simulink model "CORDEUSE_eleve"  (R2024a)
settings: Solver=VariableStepAuto  StartTime=0.0  StopTime=10.0  RelTol=1e-3
libraries: fl_lib x15, nesl_utility x4, slpidlib x1

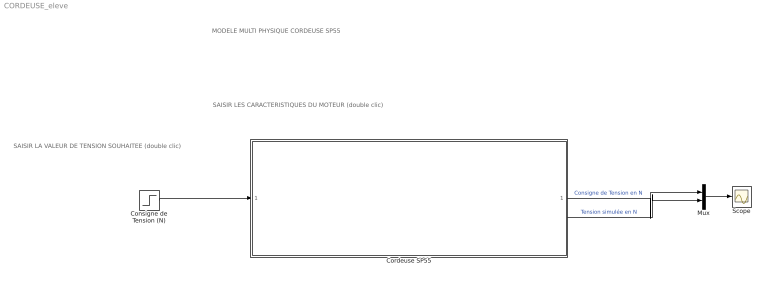
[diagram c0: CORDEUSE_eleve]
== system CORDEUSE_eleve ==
  note: MODELE MULTI PHYSIQUE CORDEUSE SP55
  note: SAISIR LES CARACTERISTIQUES DU MOTEUR (double clic)
  note: SAISIR LA VALEUR DE TENSION SOUHAITEE (double clic)
  Consigne de Tension (N) : Step  After=T  SampleTime=0.001  mask{T=4}
      mask prompts: T "Tension de consigne (en N)"
  Cordeuse SP55 : Subsystem  mask{Kc=0.0001, R=0.0001, L=0.0001}
      mask prompts: Kc "Constante de couple en N.m/A"; R "Résistance induit en ohms."; L "Inductance en mH"
  Mux : Mux  Inputs=2
  Scope : Scope
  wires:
  Mux/1 -> Scope/1
  Consigne de Tension (N)/1 -> Cordeuse SP55/1(In1)
  Cordeuse SP55/1(Consigne) -> Mux/1  "Consigne de Tension en N"
  Cordeuse SP55/2(Tension simulée) -> Mux/2  "Tension simulée en N"

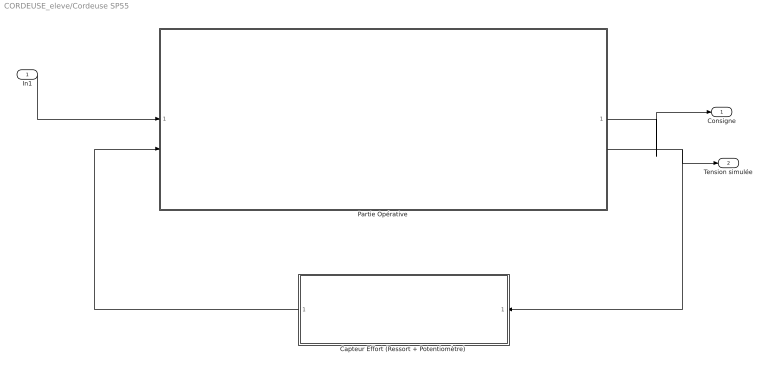
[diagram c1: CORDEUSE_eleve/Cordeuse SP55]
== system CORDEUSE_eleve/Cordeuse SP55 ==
  In1 : Inport
  Capteur Effort (Ressort + Potentiomètre) : Subsystem
  Partie Opérative : Subsystem
  Consigne : Outport
  Tension simulée : Outport  Port=2
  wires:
  Partie Opérative/2(Out2) -> Tension simulée/1, Capteur Effort (Ressort + Potentiomètre)/1(Tension simulée)
  Capteur Effort (Ressort + Potentiomètre)/1(Sortie conditionneur) -> Partie Opérative/2(In1)
  Partie Opérative/1(Out1) -> Consigne/1
  In1/1 -> Partie Opérative/1(In2)

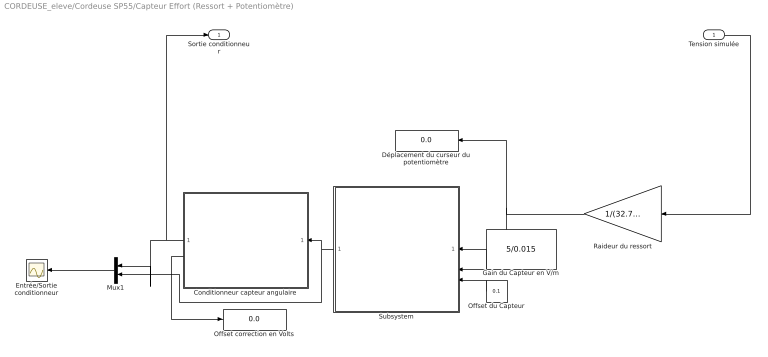
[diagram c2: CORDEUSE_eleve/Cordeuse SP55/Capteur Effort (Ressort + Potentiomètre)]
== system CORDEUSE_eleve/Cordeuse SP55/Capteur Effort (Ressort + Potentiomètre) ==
  Tension simulée : Inport
  Conditionneur capteur angulaire : Subsystem
  Déplacement du curseur du potentiomètre : Display
  Entrée/Sortie conditionneur : Scope
  Gain du Capteur en V/m : Constant  Value=5/0.015
  Mux1 : Mux  Inputs=2
  Offset correction en Volts : Display
  Offset du Capteur : Constant  Value=0.1
  Raideur du ressort : Gain  Gain=1/(32.7*1000)
  Subsystem : Subsystem
  Sortie conditionneur : Outport
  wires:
  Subsystem/1(Out1) -> Conditionneur capteur angulaire/1(Entrée capteur), Mux1/2
  Gain du Capteur en V/m/1 -> Subsystem/2(Gain du Capteur)
  Conditionneur capteur angulaire/1(Sortie conditionneur) -> Sortie conditionneur/1, Mux1/1
  Tension simulée/1 -> Raideur du ressort/1
  Conditionneur capteur angulaire/2(Offset) -> Offset correction en Volts/1
  Offset du Capteur/1 -> Subsystem/3(Offset du Capteur en Volt)
  Mux1/1 -> Entrée/Sortie conditionneur/1
  Raideur du ressort/1 -> Déplacement du curseur du potentiomètre/1, Subsystem/1(Entrée du Capteur)

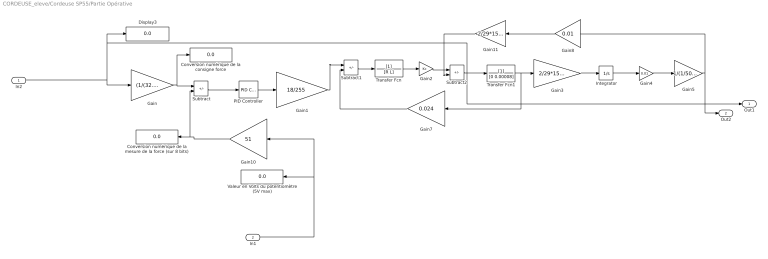
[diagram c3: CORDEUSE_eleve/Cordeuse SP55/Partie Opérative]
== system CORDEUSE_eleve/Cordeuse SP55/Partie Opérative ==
  In2 : Inport
  In1 : Inport  Port=2
  Conversion numérique de la consigne force : Display
  Conversion numérique de la mesure de la force (sur 8 bits) : Display
  Display3 : Display
  Gain : Gain  Gain=(1/(32.7*1000))*(5/0.015)*51
  Gain1 : Gain  Gain=18/255
  Gain10 : Gain  Gain=51
  Gain11 : Gain  Gain=2/29*15/55
  Gain2 : Gain  Gain=Kc
  Gain3 : Gain  Gain=2/29*15/55
  Gain4 : Gain  Gain=0.01
  Gain5 : Gain  Gain=1/(1/5052+1/(32.7*1000))
  Gain7 : Gain  Gain=0.024
  Gain8 : Gain  Gain=0.01
  Integrator : Integrator
  PID Controller : slpidlib/PID Controller  Controller=PID  Form=Parallel  TimeDomain=Continuous-time  UseExternalTs=off  SampleTime=-1  IntegratorMethod=Forward Euler  FilterMethod=Forward Euler  ControllerParametersSource=internal  P=3  I=0.4  UseKiTs=off  D=0  UseExternalDerivativeSource=off  N=100  UseFilter=on  TunerSelectOption=Transfer Function Based (PID Tuner App)  InitialConditionSource=internal  InitialConditionForIntegrator=0  InitialConditionForFilter=0  DifferentiatorICPrevScaledInput=0  ExternalReset=none  TrackingMode=off  Kt=1  LimitOutput=off  SatLimitsSource=internal  UpperSaturationLimit=inf  LowerSaturationLimit=-inf  LinearizeAsGain=on  AntiWindupMode=none  Kb=1  LimitIntegrator=off  UpperIntegratorSaturationLimit=inf  LowerIntegratorSaturationLimit=-inf  POutMin=[]  POutMax=[]  IOutMin=[]  IOutMax=[]  DOutMin=[]  DOutMax=[]  NOutMin=[]  NOutMax=[]  SumOutMin=[]  SumOutMax=[]  SaturationOutMin=[]  SaturationOutMax=[]  PParamMin=[]  PParamMax=[]  IParamMin=[]  IParamMax=[]  DParamMin=[]  DParamMax=[]  NParamMin=[]  NParamMax=[]  KbParamMin=[]  KbParamMax=[]  KtParamMin=[]  KtParamMax=[]  KbOutMin=[]  KbOutMax=[]  KtOutMin=[]  KtOutMax=[]  IntegratorOutMin=[]  IntegratorOutMax=[]  FilterOutMin=[]  FilterOutMax=[]  SumI1OutMin=[]  SumI1OutMax=[]  SumI2OutMin=[]  SumI2OutMax=[]  SumI3OutMin=[]  SumI3OutMax=[]  SumI4OutMin=[]  SumI4OutMax=[]  SumDOutMin=[]  SumDOutMax=[]  DifferentiatorOutMin=[]  DifferentiatorOutMax=[]  FilterDiffOutCoefMin=[]  FilterDiffOutCoefMax=[]  ReciprocalOutMin=[]  ReciprocalOutMax=[]  SumDenOutMin=[]  SumDenOutMax=[]  SumNumOutMin=[]  SumNumOutMax=[]  DivideOutMin=[]  DivideOutMax=[]  UdiffTsProdOutMin=[]  UdiffTsProdOutMax=[]  NTsProdOutMin=[]  NTsProdOutMax=[]  UintegralTsProdOutMin=[]  UintegralTsProdOutMax=[]  UngainTsProdOutMin=[]  UngainTsProdOutMax=[]  ClampingZeroOutDataTypeStr=Inherit: Inherit via back propagation  ClampingZeroOutMin=[]  ClampingZeroOutMax=[]  FilterDenConstantOutDataTypeStr=Inherit: Inherit via back propagation  FilterDenConstantOutMin=[]  FilterDenConstantOutMax=[]  PCopyOutDataTypeStr=Inherit: Inherit via back propagation  PCopyOutMin=[]  PCopyOutMax=[]  NCopyOutDataTypeStr=Inherit: Inherit via back propagation  NCopyOutMin=[]  NCopyOutMax=[]  IntegratorContinuousStateAttributes=''  IntegratorStateMustResolveToSignalObject=off  IntegratorRTWStateStorageClass=Auto  FilterContinuousStateAttributes=''  FilterStateMustResolveToSignalObject=off  FilterRTWStateStorageClass=Auto  ParallelPVariant=InternalParameters  IdealPVariant=Disabled  IVariant=InternalParameters  DVariant=InternalParameters  IntegratorVariant=Continuous  SatVariant=Disabled  AWVariant=Passthrough  PCopyVariant=Disabled  TRVariant=Disabled  FdbkBlocksVariant=Forward  IdealPFdbkVariant=Disabled  SatFdbkVariant=Disabled  DerivativeFilterVariant=ContFilter  NVariant=InternalParameters  NCopyVariant=Disabled  FilterICVariant=InternalICsFilter  IntegratorICVariant=InternalICs  ExternalResetVariant=Disabled  TRSumVariant=Passthrough  SumFdbkVariant=Disabled  SumVariant=Sum_PID  TsampFilterVariant=InternalTs  TsampNgainVariant=Passthrough  TsampIntegralVariant=Disabled_SignalSpec  ExternalSaturationOutDataTypeStr=Inherit: Same as second input  DerivativeSourceVariant=ErrorSignal
  Subtract : Sum  Inputs=+-
  Subtract1 : Sum  Inputs=+-
  Subtract2 : Sum  Inputs=+-
  Transfer Fcn : TransferFcn  Denominator=[R L]
  Transfer Fcn1 : TransferFcn  Denominator=[0 0.00008]
  Valeur en Volts du potentiomètre (5V max) : Display
  Out1 : Outport
  Out2 : Outport  Port=2
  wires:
  PID Controller/1 -> Gain1/1
  Integrator/1 -> Gain4/1
  Gain/1 -> Conversion numérique de la consigne force/1, Subtract/1
  In2/1 -> Gain/1, Display3/1, Out1/1
  Gain5/1 -> Out2/1, Gain8/1
  Subtract/1 -> PID Controller/1
  Transfer Fcn1/1 -> Gain7/1, Gain3/1
  Subtract1/1 -> Transfer Fcn/1
  Transfer Fcn/1 -> Gain2/1
  Gain10/1 -> Subtract/2, Conversion numérique de la mesure de la force (sur 8 bits)/1
  In1/1 -> Valeur en Volts du potentiomètre (5V max)/1, Gain10/1
  Subtract2/1 -> Transfer Fcn1/1
  Gain4/1 -> Gain5/1
  Gain2/1 -> Subtract2/1
  Gain3/1 -> Integrator/1
  Gain11/1 -> Subtract2/2
  Gain1/1 -> Subtract1/1
  Gain7/1 -> Subtract1/2
  Gain8/1 -> Gain11/1

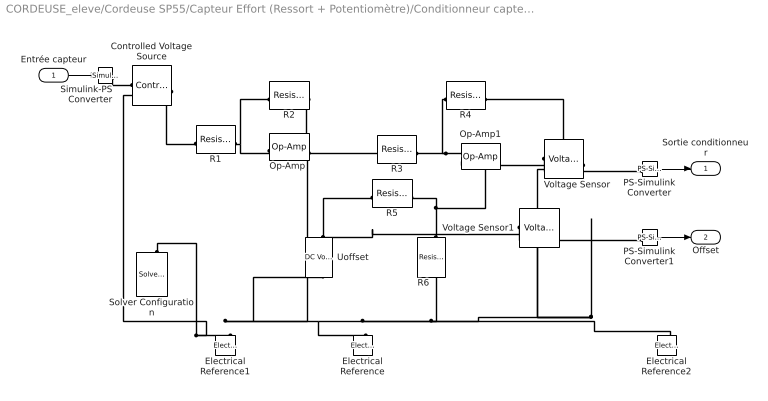
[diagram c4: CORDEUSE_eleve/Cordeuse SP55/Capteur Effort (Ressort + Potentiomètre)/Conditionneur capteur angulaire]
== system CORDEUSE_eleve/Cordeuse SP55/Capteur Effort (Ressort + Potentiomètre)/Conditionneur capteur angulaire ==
  Entrée capteur : Inport
  Controlled Voltage Source : fl_lib/Electrical/Electrical Sources/Controlled Voltage Source
  Electrical Reference : fl_lib/Electrical/Electrical Elements/Electrical Reference
  Electrical Reference1 : fl_lib/Electrical/Electrical Elements/Electrical Reference
  Electrical Reference2 : fl_lib/Electrical/Electrical Elements/Electrical Reference
  Op-Amp : fl_lib/Electrical/Electrical Elements/Op-Amp  outI_specify=off  outI_priority=None  outI=0 A  outI_nominal_specify=off  outI_nominal_value=1  outI_nominal_unit=A
  Op-Amp1 : fl_lib/Electrical/Electrical Elements/Op-Amp  outI_specify=off  outI_priority=None  outI=0 A  outI_nominal_specify=off  outI_nominal_value=1  outI_nominal_unit=A
  PS-Simulink Converter : nesl_utility/PS-Simulink Converter  PhysicalDomain=network_engine_domain  SubClassName=ps_output  LeftPortType=input  RightPortType=output  PseudoPeriodic=off  Frequencies=[]  VectorFormat=inherit  Unit=inherit  AffineConversion=off
  PS-Simulink Converter1 : nesl_utility/PS-Simulink Converter  PhysicalDomain=network_engine_domain  SubClassName=ps_output  LeftPortType=input  RightPortType=output  PseudoPeriodic=off  Frequencies=[]  VectorFormat=inherit  Unit=inherit  AffineConversion=off
  R1 : fl_lib/Electrical/Electrical Elements/Resistor  R=1 Ohm  i_specify=off  i_priority=None  i=0 A  i_nominal_specify=off  i_nominal_value=1  i_nominal_unit=A  v_specify=off  v_priority=None  v=0 V  v_nominal_specify=off  v_nominal_value=1  v_nominal_unit=V
  R2 : fl_lib/Electrical/Electrical Elements/Resistor  R=2 Ohm  i_specify=off  i_priority=None  i=0 A  i_nominal_specify=off  i_nominal_value=1  i_nominal_unit=A  v_specify=off  v_priority=None  v=0 V  v_nominal_specify=off  v_nominal_value=1  v_nominal_unit=V
  R3 : fl_lib/Electrical/Electrical Elements/Resistor  R=10 Ohm  i_specify=off  i_priority=None  i=0 A  i_nominal_specify=off  i_nominal_value=1  i_nominal_unit=A  v_specify=off  v_priority=None  v=0 V  v_nominal_specify=off  v_nominal_value=1  v_nominal_unit=V
  R4 : fl_lib/Electrical/Electrical Elements/Resistor  R=5 Ohm  i_specify=off  i_priority=None  i=0 A  i_nominal_specify=off  i_nominal_value=1  i_nominal_unit=A  v_specify=off  v_priority=None  v=0 V  v_nominal_specify=off  v_nominal_value=1  v_nominal_unit=V
  R5 : fl_lib/Electrical/Electrical Elements/Resistor  R=11 Ohm  i_specify=off  i_priority=None  i=0 A  i_nominal_specify=off  i_nominal_value=1  i_nominal_unit=A  v_specify=off  v_priority=None  v=0 V  v_nominal_specify=off  v_nominal_value=1  v_nominal_unit=V
  R6 : fl_lib/Electrical/Electrical Elements/Resistor  R=13 Ohm  i_specify=off  i_priority=None  i=0 A  i_nominal_specify=off  i_nominal_value=1  i_nominal_unit=A  v_specify=off  v_priority=None  v=0 V  v_nominal_specify=off  v_nominal_value=1  v_nominal_unit=V
  Simulink-PS Converter : nesl_utility/Simulink-PS Converter  PhysicalDomain=network_engine_domain  SubClassName=ps_input  LeftPortType=input  RightPortType=output  PseudoPeriodic=off  Frequencies=[]  NoiseDistribution=none  NoiseParameters=[]  Unit=1  AffineConversion=off  FilteringAndDerivatives=provide  SimscapeFilterOrder=1  InputFilterTimeConstant=0.001  UdotUserProvided=0
  Solver Configuration : nesl_utility/Solver Configuration  PhysicalDomain=network_engine_domain  SubClassName=solver  LeftPortType=input  RightPortType=generic  Tones=[]  Harmonics=[]  SimulateNoise=off  Profile=off  UseLocalSampling=off  EnableSwitchedLinearOptims=on  FrequencyDomain=off  UseCCode=off  RelTol=0.001  AbsTol=0.001  MinStep=1e-09  ToWorkspace=off  RevertToSquareIcSolve=off  NumHomotopyIterations=100  PhasorMode=off  PhasorModeNumHarmonics=1  ConsistencySolver=NEWTON_FTOL  IndexReductionMethod=DerivativeReplacement  DoDC=off  ResidualTolerance=1e-09  ConsistencyTolSource=GLOBAL  ConsistencyAbsTol=0.001  ConsistencyRelTol=0.001  ConsistencyTolFactor=0.001  UseLocalSolver=off  LocalSolverChoice=NE_BACKWARD_EULER_ADVANCER  ResolveIndetEquations=on  FunctionEvalNumThread=1  LocalSolverSampleTime=0.001  DoFixedCost=off  MaxNonlinIter=3  MaxModeIter=2  ComputeImpulses=off  ImpulseIterations=2  LinearAlgebra=auto  LinearAlgebraNumThread=0  EquationFormulation=NE_TIME_EF  DelaysMemoryBudget=1024  AutomaticFiltering=on  FilteringTimeConstant=0.001  PartitionStorageMethod=AS_NEEDED  PartitionMemoryBudget=1024  PartitionMethod=ROBUST  MultibodyUseLocalSolver=off  MultibodyLocalSolverChoice=ODE1  MultibodyLocalSolverSampleTime=0.001
  Uoffset : fl_lib/Electrical/Electrical Sources/DC Voltage Source  v0=-0.1 V
  Voltage Sensor : fl_lib/Electrical/Electrical Sensors/Voltage Sensor
  Voltage Sensor1 : fl_lib/Electrical/Electrical Sensors/Voltage Sensor
  Sortie conditionneur : Outport
  Offset : Outport  Port=2
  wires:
  PS-Simulink Converter/1 -> Sortie conditionneur/1
  Entrée capteur/1 -> Simulink-PS Converter/1
  PS-Simulink Converter1/1 -> Offset/1
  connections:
  Solver Configuration/RConn1 -- Voltage Sensor1/RConn2 -- Voltage Sensor/RConn2 -- Electrical Reference2/LConn1 -- R6/RConn1 -- Electrical Reference/LConn1 -- Uoffset/RConn1 -- Op-Amp/LConn1 -- Electrical Reference1/LConn1 -- Controlled Voltage Source/RConn2
  Voltage Sensor/RConn1 -- PS-Simulink Converter/LConn1
  Simulink-PS Converter/RConn1 -- Controlled Voltage Source/RConn1
  Controlled Voltage Source/LConn1 -- R1/LConn1
  R1/RConn1 -- R2/LConn1 -- Op-Amp/LConn2
  R2/RConn1 -- R3/LConn1 -- Op-Amp/RConn1
  R4/LConn1 -- Op-Amp1/LConn2 -- R3/RConn1
  Voltage Sensor/LConn1 -- Op-Amp1/RConn1 -- R4/RConn1
  Voltage Sensor1/RConn1 -- PS-Simulink Converter1/LConn1
  Uoffset/LConn1 -- R5/LConn1 -- Voltage Sensor1/LConn1
  R6/LConn1 -- Op-Amp1/LConn1 -- R5/RConn1

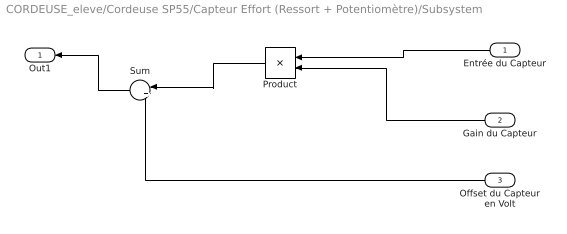
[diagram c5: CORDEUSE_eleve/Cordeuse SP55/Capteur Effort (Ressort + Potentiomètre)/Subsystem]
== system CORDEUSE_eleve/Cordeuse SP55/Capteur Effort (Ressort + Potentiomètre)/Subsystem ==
  Entrée du Capteur : Inport
  Gain du Capteur : Inport  Port=2
  Offset du Capteur en Volt : Inport  Port=3
  Product : Product
  Sum : Sum  Inputs=|++
  Out1 : Outport
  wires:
  Sum/1 -> Out1/1
  Product/1 -> Sum/1
  Entrée du Capteur/1 -> Product/1
  Offset du Capteur en Volt/1 -> Sum/2
  Gain du Capteur/1 -> Product/2
